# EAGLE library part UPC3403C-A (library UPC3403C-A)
Support is limited to customers who have already adopted these products. Source: Datasheet
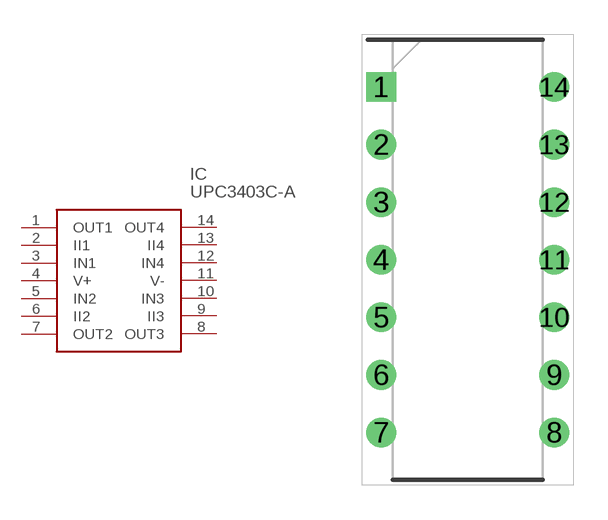
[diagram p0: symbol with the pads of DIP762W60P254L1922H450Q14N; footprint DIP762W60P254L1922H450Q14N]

Designator prefix IC

## UPC3403C-A (Description: Support is limited to customers who have already adopted these products.; Height: 4.5mm; Manufacturer_Name: Renesas Electronics; Manufacturer_Part_Number: UPC3403C-A)  [DIP762W60P254L1922H450Q14N]
1  OUT1
2  II1
3  IN1
4  V+
5  IN2
6  II2
7  OUT2
8  OUT3
9  II3
10  IN3
11  V-
12  IN4
13  II4
14  OUT4

## Footprint DIP762W60P254L1922H450Q14N (pad centres in mm)
14-PIN PLASTIC TSSOP (5.72mm (225))
drill 0.8 pad 1.2 square: 1 -3.81,7.62
drill 0.8 pad 1.2: 2 -3.81,5.08; 3 -3.81,2.54; 4 -3.81,0; 5 -3.81,-2.54; 6 -3.81,-5.08; 7 -3.81,-7.62; 8 3.81,-7.62; 9 3.81,-5.08; 10 3.81,-2.54; 11 3.81,0; 12 3.81,2.54; 13 3.81,5.08; 14 3.81,7.62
